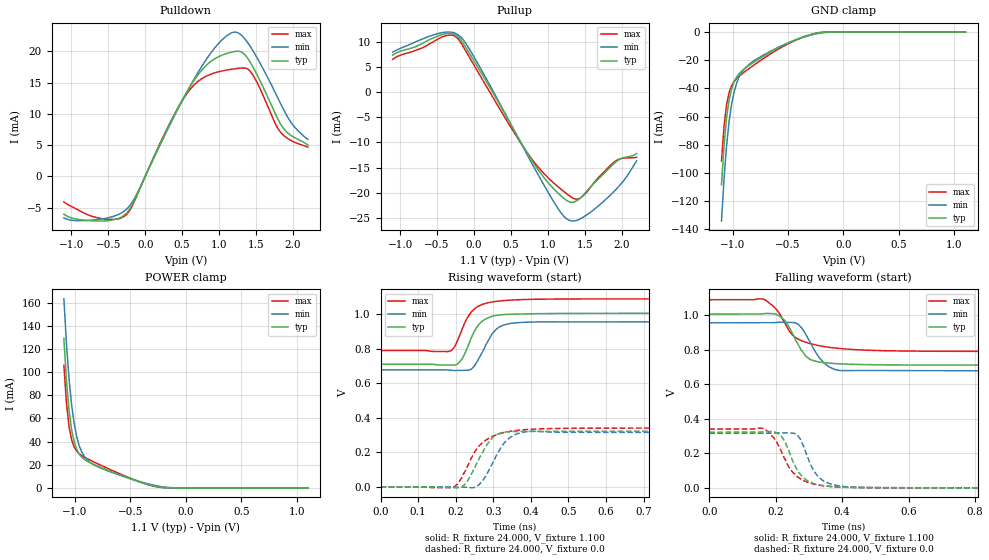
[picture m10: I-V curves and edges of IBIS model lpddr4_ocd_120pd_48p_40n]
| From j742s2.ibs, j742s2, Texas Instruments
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|   Model lpddr4_ocd_120pd_48p_40n
[Model] lpddr4_ocd_120pd_48p_40n
Model_type I/O
Polarity   Non-Inverting
Enable   Active-High
Vinl =  0.113V
Vinh =  0.253V
Vmeas =  0.183V
C_comp   1.400pF   1.229pF   1.662pF
[Model Spec]
Vinh   0.253V   0.247V   0.265V
Vinl   0.113V   0.107V   0.125V
Vmeas   0.183V   0.176V   0.195V
[Temperature Range]   25.000   0.125k   -40.000
[Voltage Range]   1.100V   1.060V   1.170V
[Pullup Reference]   1.100V   1.060V   1.170V
[Pulldown Reference]   0.0V   0.0V   0.0V
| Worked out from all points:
|   slope of the pulldown table from 0 to 0.165 V, typ, clamps not added: 38.6 ohm
|   slope of the pullup table from 0 to 0.165 V, typ, clamps not added: 40.7 ohm
|   GND clamp passes 1 mA (typ) near -0.25 V on its own axis
|   POWER clamp passes 1 mA (typ) near -0.26 V on its own axis
|   rising waveform, R_fixture 24.000, V_fixture 1.100: 20-80 % time 40.3ps typ, 43ps min, 44ps max; typ from 0.71 V to 1.01 V
|   rising waveform, R_fixture 24.000, V_fixture 0.0: 20-80 % time 48.6ps typ, 48.5ps min, 62.4ps max; typ from 0 V to 0.322 V
|   falling waveform, R_fixture 24.000, V_fixture 1.100: 20-80 % time 52.9ps typ, 53ps min, 76.8ps max; typ from 1.01 V to 0.71 V
|   falling waveform, R_fixture 24.000, V_fixture 0.0: 20-80 % time 50ps typ, 48ps min, 62.6ps max; typ from 0.322 V to 0 V
[Pulldown]
|Voltage   I(typ)   I(min)   I(max)
-1.1V     -6.056mA   -6.655mA   -4.075mA
-658mV    -7.127mA   -6.914mA   -6.588mA
-284mV    -6.208mA   -5.549mA   -6.391mA
-113mV    -2.983mA   -2.787mA   -3.073mA
295mV     7.517mA    7.322mA    7.636mA
567mV     13.62mA    13.58mA    13.31mA
839mV     17.92mA    18.95mA    16.13mA
1.179V    19.93mA    23.04mA    17.18mA
1.418V    18.32mA    20.86mA    16.88mA
1.826V    8.488mA    11.79mA    7.15mA
1.996V    6.386mA    8.257mA    5.615mA
2.2V      5.031mA    5.92mA     4.7mA
[Pullup]
|Voltage   I(typ)   I(min)   I(max)
-1.1V     7.385mA    7.991mA    6.542mA
-386mV    11.65mA    11.96mA    11.23mA
-284mV    11.63mA    11.88mA    11.32mA
-181mV    10.46mA    11.02mA    9.921mA
90.72mV   3.992mA    4.686mA    3.087mA
737mV     -12.52mA   -12.94mA   -12.41mA
1.111V    -19.73mA   -22.58mA   -18.51mA
1.281V    -21.8mA    -25.46mA   -20.53mA
1.452V    -20.88mA   -25.11mA   -20.94mA
1.724V    -16.67mA   -22.12mA   -16.38mA
1.928V    -13.77mA   -19.23mA   -13.57mA
2.2V      -12.22mA   -13.66mA   -12.97mA
[GND_clamp]
|Voltage   I(typ)   I(min)   I(max)
-1.1V     -108.4mA   -134.2mA   -91.64mA
-1.077V   -80.17mA   -103.9mA   -66.64mA
-1.054V   -60.68mA   -80.47mA   -51.43mA
-1.031V   -48.01mA   -63.16mA   -42.83mA
-1.008V   -40.05mA   -50.75mA   -37.97mA
-985mV    -35.04mA   -42.04mA   -34.98mA
-940mV    -29.42mA   -31.64mA   -31.22mA
-894mV    -26.11mA   -26.16mA   -28.35mA
-848mV    -23.5mA    -22.73mA   -25.7mA
-527mV    -8.739mA   -8.686mA   -9.515mA
-229mV    -630.6uA   -1.042mA   -565.6uA
1.1V      0A         0A         0A
[POWER_clamp]
|Voltage   I(typ)   I(min)   I(max)
-1.1V     129.2mA    163.4mA    105.9mA
-1.077V   92.86mA    124.8mA    73.4mA
-1.054V   67.3mA     94.73mA    53.17mA
-1.031V   50.48mA    72.25mA    41.67mA
-1.008V   39.92mA    56.03mA    35.37mA
-985mV    33.38mA    44.6mA     31.76mA
-963mV    29.31mA    36.69mA    29.53mA
-917mV    24.75mA    27.38mA    26.61mA
-871mV    22.09mA    22.57mA    24.31mA
-619mV    11.98mA    11.76mA    13.12mA
-229mV    602.6uA    1.183mA    400.6uA
1.1V      0A         0A         0A
[Ramp]
| variable   typ   min   max
dV/dt_r   0.259/52.852p   0.250/51.958p   0.280/72.712p
dV/dt_f   0.249/60.505p   0.229/58.424p   0.272/0.106n
R_load = 40.000
[Rising Waveform]
R_fixture= 24.000
V_fixture= 1.100
V_fixture_min= 1.060
V_fixture_max= 1.170
|time   V(typ)   V(min)   V(max)
0s        710.5mV    678mV      790.1mV
185ps     706.7mV    676mV      786.8mV
199ps     707mV      674.3mV    818.4mV
210ps     721.3mV    675mV      875.6mV
238ps     843.8mV    678.4mV    1.003V
267ps     954.1mV    765.3mV    1.054V
296ps     987.4mV    884.9mV    1.071V
310ps     994.4mV    917.5mV    1.076V
364ps     1.002V     951.5mV    1.084V
3ns       1.006V     956mV      1.09V
[Rising Waveform]
R_fixture= 24.000
V_fixture= 0.0
V_fixture_min= 0.0
V_fixture_max= 0.0
|time   V(typ)   V(min)   V(max)
0s        129.4uV    208.6uV    249uV
193ps     -3.995mV   -3.119mV   -3.117mV
208ps     -4.508mV   -2.601mV   24.66mV
220ps     4.079mV    -2mV       71.09mV
251ps     112mV      -3.038mV   203.8mV
279ps     229.2mV    57.69mV    268.9mV
307ps     300.8mV    176.7mV    300.6mV
343ps     319.5mV    283.7mV    321.2mV
399ps     321.4mV    321.4mV    333.7mV
3ns       322.4mV    315.9mV    340.6mV
[Falling Waveform]
R_fixture= 24.000
V_fixture= 1.100
V_fixture_min= 1.060
V_fixture_max= 1.170
|time   V(typ)   V(min)   V(max)
0s        1.006V     956mV      1.09V
164ps     1.009V     956mV      1.092V
199ps     1.006V     957.7mV    1.04V
219ps     984.4mV    959mV      982.6mV
261ps     851.9mV    954.6mV    868.2mV
277ps     798mV      929.6mV    852.2mV
301ps     745.8mV    852.3mV    836.7mV
341ps     726.1mV    731.7mV    819.7mV
386ps     718.8mV    682.7mV    808.2mV
3ns       710.5mV    678mV      790.1mV
[Falling Waveform]
R_fixture= 24.000
V_fixture= 0.0
V_fixture_min= 0.0
V_fixture_max= 0.0
|time   V(typ)   V(min)   V(max)
0s        322.3mV    315.9mV    340.6mV
167ps     326.1mV    315.9mV    340.9mV
199ps     322.6mV    317.7mV    278.2mV
219ps     294.1mV    319.1mV    202.7mV
256ps     135.2mV    315.7mV    80.37mV
273ps     80.88mV    286.2mV    55.04mV
321ps     21.66mV    81.34mV    19.02mV
374ps     6.516mV    18.3mV     6.408mV
538ps     763.9uV    810.9uV    994.1uV
3ns       128.4uV    207.9uV    248.9uV
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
